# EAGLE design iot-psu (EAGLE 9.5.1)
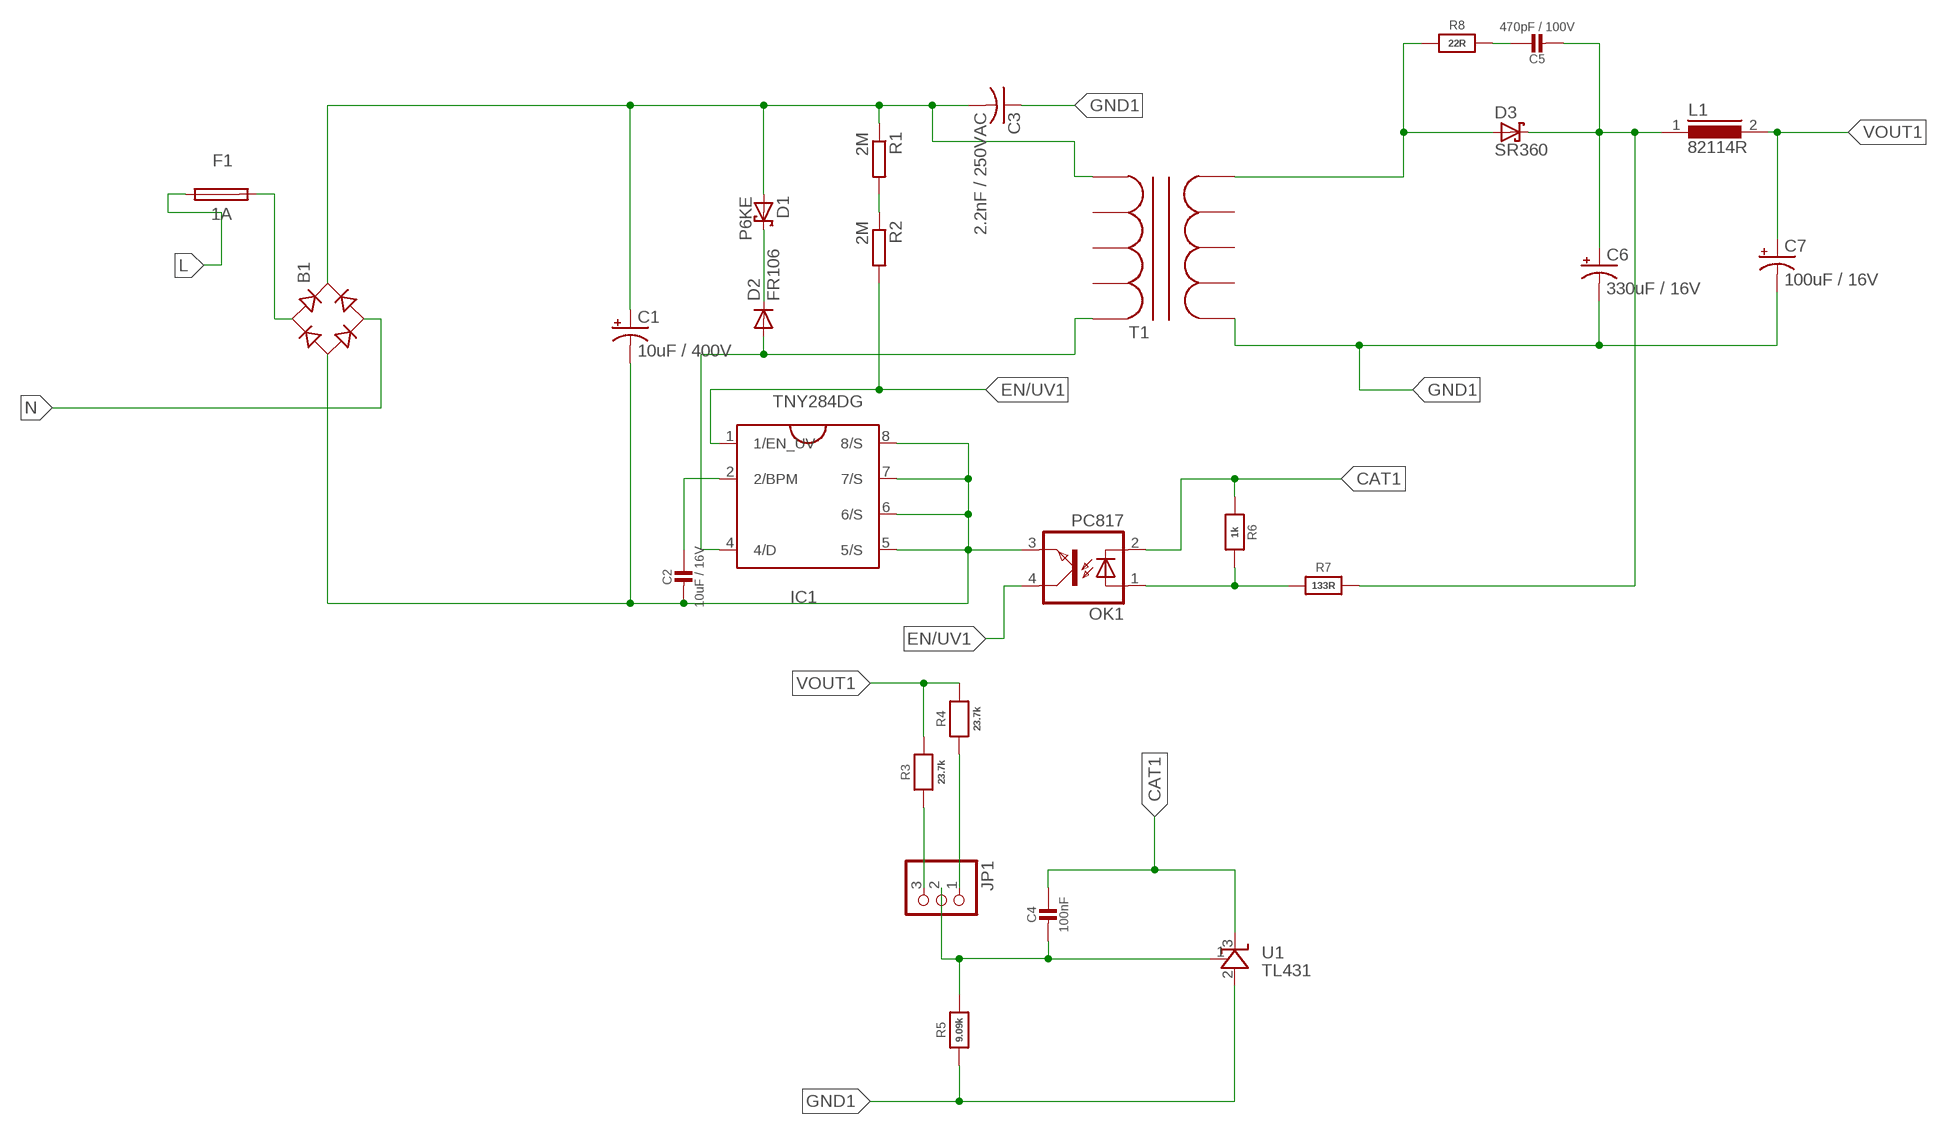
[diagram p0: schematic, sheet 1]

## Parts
B1  B-DIL  [B-DIL]
C1  10uF / 400V  CPOL-USE5-10.5  [E5-10,5]
C2  10uF / 16V  CAP_CERAMIC0805-NOOUTLINE  [0805-NO]
C3  2.2nF / 250VAC  C-US075-032X103  [C075-032X103]
C4  100nF  CAP_CERAMIC0805-NOOUTLINE  [0805-NO]
C5  470pF / 100V  CAP_CERAMIC0805-NOOUTLINE  [0805-NO]
C6  330uF / 16V  CPOL-USE3.5-8  [E3,5-8]
C7  100uF / 16V  CPOL-USE2.5-7  [E2,5-7]
D1  P6KE  P6KEXX  [CB417-15]
D2  FR106  1N4004  [DO41-10]
D3  SR360  SCHOTTKY-DIODEC4111-15  [C4111-15]
F1  1A  TR5  [TR5]
IC1  TNY284DG  TNY375-380SO8-C  [SO8-C(D_PACKAGE)]
JP1  PINHD-1X3  [1X03]
L1  82114R  [82114R]
OK1  PC817  [DIL04]
R1  2M  R-EU_M1206  [M1206]
R2  2M  R-EU_M1206  [M1206]
R3  23.7k  RESISTOR0805_NOOUTLINE  [0805-NO]
R4  23.7k  RESISTOR0805_NOOUTLINE  [0805-NO]
R5  9.09k  RESISTOR0805_NOOUTLINE  [0805-NO]
R6  1k  RESISTOR0805_NOOUTLINE  [0805-NO]
R7  133R  RESISTOR0805_NOOUTLINE  [0805-NO]
R8  22R  RESISTOR0805_NOOUTLINE  [0805-NO]
T1  TRANSFORMER_EE16  [EE16]
U1  TL431  [TO-92]

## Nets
AN1: C5.2 C6.+ D3.C L1.1 R7.2
BP/M: C2.1 IC1.2(2/BPM)
CAT1: C4.1 OK1.2(C) R6.1 U1.3(C)
DRAIN: D2.A IC1.4(4/D) T1.P$5
EN/UV1: IC1.1(1/EN_UV) OK1.4(COL) R2.2
GND1: C3.1 C6.- C7.- R5.1 T1.P$6 U1.2(A)
HV+: B1.+ C1.+ C3.2 D1.A R1.1 T1.P$1
L: F1.P$1
N: B1.AC2
N$1: JP1.1 R4.1
N$2: JP1.3 R3.1
N$5: OK1.1(A) R6.2 R7.1
N$6: D1.C D2.C
N$7: C5.1 R8.2
N$9: R1.2 R2.1
N$13: C4.2 JP1.2 R5.2 U1.1(REF)
N$50: B1.AC1 F1.P$2
SEC1: D3.A R8.1 T1.P$10
SOURCE: B1.- C1.- C2.2 IC1.5(5/S) IC1.6(6/S) IC1.7(7/S) IC1.8(8/S) OK1.3(EMIT)
VOUT1: C7.+ L1.2 R3.2 R4.2
Unconnected: T1.P$2 T1.P$3 T1.P$4 T1.P$7 T1.P$8 T1.P$9

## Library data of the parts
B1 = rectifier:B-DIL: RECTIFIER
C1 C6 C7 = resistor:CPOL-US: POLARIZED CAPACITOR, American symbol
C2 C4 C5 = microbuilder:CAP_CERAMIC: Ceramic Capacitors
C3 = resistor:C-US: CAPACITOR, American symbol
D1 = NRG Lib:P6KEXX: DIODE
D2 = NRG Lib:1N4004: DIODE
D3 = NRG Lib:SCHOTTKY-DIODE: Schottky Diode
F1 = nrg_single:TR5: FUSE
IC1 = power_integrations:TNY375-380: TinySwitch-PK incorporates a 700 V MOSFET, oscillator, highvoltage switched current source, current limit (user selectable), and thermal shutdown circuitry. A unique peak mode feature boosts current limit and frequency for peak load conditions. The boosted current limit provides the peak output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
JP1 = pinhead:PINHD-1X3: PIN HEADER
L1 = inductors:82114R: INDUCTOR
OK1 = NRG Lib:PC817: SHARP OPTO COUPLER; MPN: PC817X4J000F; OC_FARNELL: 9707727; OC_NEWARK: 97K7059
R1 R2 = resistor:R-EU_: RESISTOR, European symbol
R3-R8 = microbuilder:RESISTOR: Resistors
T1 = nrg_iso_rhythm:TRANSFORMER_EE16
U1 = NRG Lib:TL431

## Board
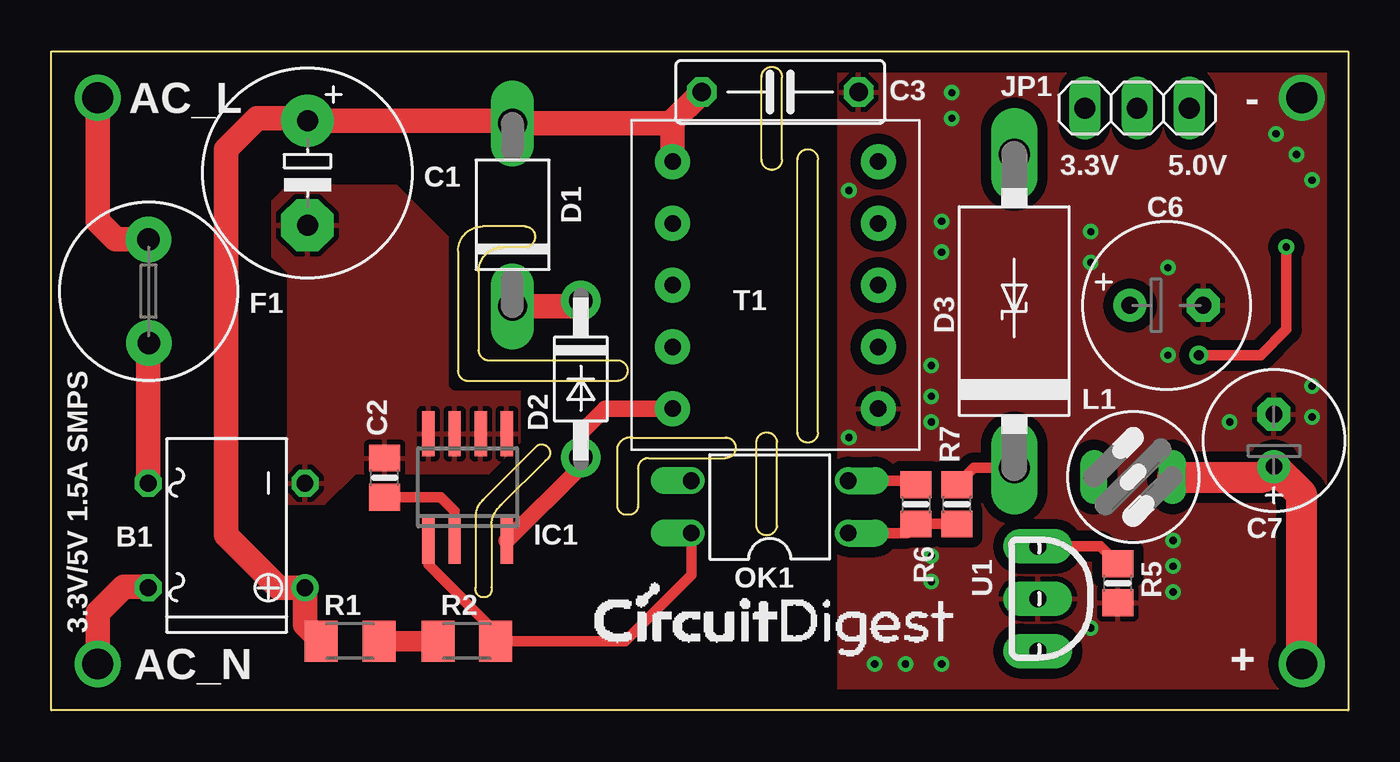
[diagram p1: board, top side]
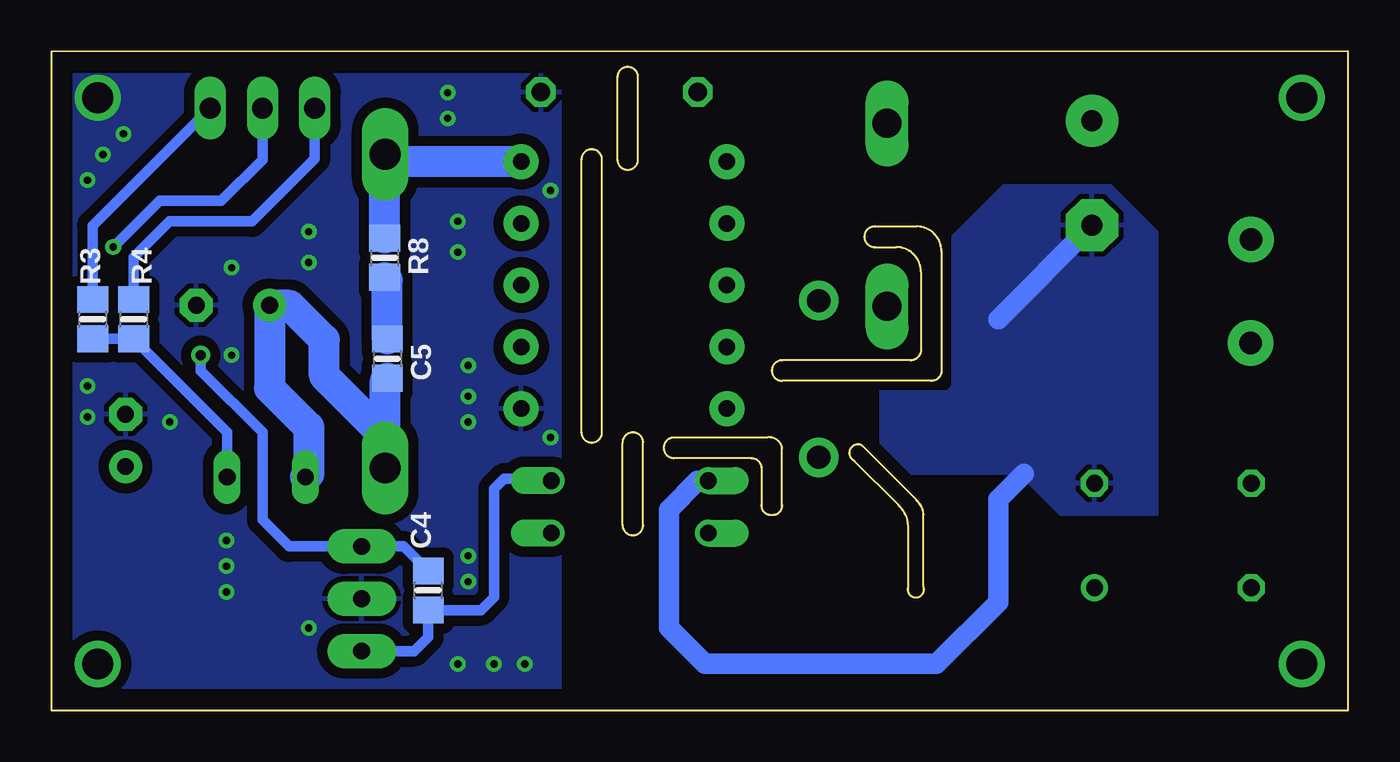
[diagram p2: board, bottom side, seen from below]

Size 63 x 32 mm. Coordinates in mm from the lower left corner, seen from the top.
Outline: 0,0 63,0 63,32 0,32 0,0
Copper layers (1*16): Top 0.035mm / dielectric 1.5mm / Bottom 0.035mm
Design rules "default *": minimum track width 6mil, minimum drill 0.35mm, track to track 0.35mm, track to pad 0.35mm, pad to pad 0.35mm, via to via 0.35mm, smd to smd 6mil, copper to edge 40mil, drill to drill 6mil, minimum pad ring 10mil, minimum via ring 8mil, stop-mask expansion 4mil, vias tented up to drill 0.5mm, thermal gap 10mil
Milling: 48 lines

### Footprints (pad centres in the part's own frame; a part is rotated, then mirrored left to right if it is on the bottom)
B-DIL = drill 0.813: + -2.54,-3.81 | drill 0.813 octagon: - 2.54,-3.81; AC1 2.54,3.81; AC2 -2.54,3.81
E5-10,5 = drill 1.016 pad 2.54: + -2.54,0 | drill 1.016 pad 2.54 octagon: - 2.54,0
0805-NO = smd 1.3 x 1.5: 1 -0.95,0; 2 0.95,0
C075-032X103 = drill 0.914 octagon: 1 -3.81,0; 2 3.81,0
E3,5-8 = drill 0.813 pad 1.6: + -1.778,0 | drill 0.813 pad 1.6 octagon: - 1.778,0
E2,5-7 = drill 0.813 pad 1.6: + -1.27,0 | drill 0.813 pad 1.6 octagon: - 1.27,0
CB417-15 = drill 1.397 long: A 2.54,0; C -6.35,0
DO41-10 = drill 1.118 pad 1.93: A 3.81,0; C -3.81,0
C4111-15 = drill 1.499 long: A 7.62,0; C -7.62,0
TR5 = drill 1.1 pad 2.2: P$1 -2.52,-0.01; P$2 2.51,0.02
SO8-C(D_PACKAGE) = smd 0.6 x 2.2: 1 -1.905,-2.6; 2 -0.635,-2.6; 4 1.905,-2.6; 5 1.905,2.6; 6 0.635,2.6; 7 -0.635,2.6; 8 -1.905,2.6
1X03 = drill 1.016 long: 1 -2.54,0; 2 0,0; 3 2.54,0
82114R = drill 0.813 long: 1 0,1.905; 2 0,-1.905
DIL04 = drill 0.813 offset: 1 -1.27,-3.81; 2 1.27,-3.81; 3 1.27,3.81; 4 -1.27,3.81
M1206 = smd 1.6 x 2: 1 -1.4,0; 2 1.4,0
EE16 = drill 0.8 pad 1.7: P$1 -6,-5; P$2 -3,-5; P$3 0,-5; P$4 3,-5; P$5 6,-5; P$6 6,5; P$7 3,5; P$8 0,5; P$9 -3,5; P$10 -6,5
TO-92 = drill 0.813 pad 1.676 long: 1 -2.54,0.318; 2 0,0.318; 3 2.54,0.318

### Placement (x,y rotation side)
B1  8.51,8.49 90 top
C1  12.44,26.1 270 top
C2  16.18,11.3 90 top
C3  35.41,30.03 180 top
C4  44.69,5.82 90 bottom
C5  46.68,17.08 270 bottom
C6  54.18,19.67 0 top
C7  59.4,13.11 90 top
D1  22.4,25.97 90 top
D2  25.72,16.09 270 top
D3  46.78,19.39 90 top
F1  4.72,20.35 270 top
IC1  20.22,10.83 0 top
JP1  52.75,29.25 0 top
L1  52.56,11.33 90 top
OK1  34.9,9.88 90 top
R1  14.51,3.36 0 top
R2  20.18,3.36 0 top
R3  61,19 270 bottom
R4  59,19 270 bottom
R5  51.81,6.17 90 top
R6  42,10 270 top
R7  44,10 90 top
R8  46.81,21.98 270 bottom
T1  35.18,20.65 270 top
U1  47.61,5.42 270 top

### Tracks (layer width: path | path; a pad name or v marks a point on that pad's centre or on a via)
AN1
  Top 0.5: R7.2 44.82,11.77 D3.C
  Bottom 1.5: L1.1 50.5,11.48 50.5,13.75 52.4,15.65 C6.+ 51.42,19.67 49.75,18 49.75,16.25 46.78,13.28 D3.C 46.78,16.03 C5.2
BP/M
  Top 0.5: IC1.2 19.59,9.66 18.9,10.35 C2.1
CAT1
  Top 0.5: OK1.2 41.8,11.15 R6.1
  Bottom 0.5: U1.3 45.37,2.88 44.69,3.56 C4.1 42.13,4.87 41.5,5.5 41.5,10.75 41,11.25 38.81,11.25 OK1.2
DRAIN
  Top 0.8: IC1.4 25.72,11.82 D2.A 25.72,13.47 26.9,14.65 T1.P$5
EN/UV1
  Top 0.5: IC1.1 18.32,7.07 21.58,3.8 R2.2 27.86,3.36 31.09,6.59 OK1.4
GND1  (via drill 0.35, 1.5)
  other vias: 60.75,29.75 42.75,16.75 42.75,15.25 42.75,14 50.5,4 43.25,2.25 41.5,2.25 40,2.25 38.75,13.25 42.75,6.25 42.75,7.5 54.5,8.25 54.5,7 54.5,5.75 61.25,14.25 61.25,15.75 57.25,14 54.25,17.25 54.25,21.5 50.5,23.25 50.5,21.75 43.25,23.75 43.25,22.25 59.5,28 60.5,27 61.25,25.75 43.75,30 43.75,28.75 38.75,25.25
  pour Bottom (isolate 0.5, rank 5): 38.25,31.5 62.5,31.5 62.5,0.5 38.25,0.5
  pour Top (isolate 0.5, rank 5): 38.25,31.5 62.5,31.5 62.5,1 38.25,1
HV+
  Top 1.2: R1.1 12.32,4.15 B1.+ 11.05,5.95 8.5,8.5 8.5,27.25 10,28.75 12.33,28.75 C1.+ 22.27,28.64 D1.A 30.08,28.51 | 30.08,28.51 C3.2 | T1.P$1 30.18,28.41 30.08,28.51
L  (via drill 1.5)
  Top 1.2: F1.P$1 3.13,22.87 2.25,23.75 v2.25,29.75
N  (via drill 1.5)
  Top 1.2: v2.25,2.25 2.25,4.75 3.5,6 4.65,6 B1.AC2
N$1
  Bottom 0.5: JP1.1 50.21,26.79 53.25,23.75 57.25,23.75 59,22 R4.1
N$2
  Bottom 0.5: JP1.3 61,23.54 R3.1
N$5
  Top 0.5: OK1.1 41.56,8.61 R6.2 R7.1
N$6
  Top 1.2: D1.C 25.44,19.62 D2.C
N$7
  Bottom 1.5: C5.1 46.68,20.9 R8.2
N$9
  Top 1: R1.2 R2.1
N$13  (via drill 0.35, 0.5)
  Top 0.5: R5.2 50.97,7.96 U1.1 | v55.75,17.25 58.75,17.25 60,18.5 v60,22.5
  Bottom 0.5: C4.2 45.88,7.96 U1.1 51.46,7.96 52.75,9.25 52.75,13.5 55.75,16.5 v55.75,17.25 | v60,22.5 57.75,24.75 54.75,24.75 52.75,26.75 JP1.2
N$50
  Top 1.2: B1.AC1 4.7,17.8 F1.P$2
SEC1
  Bottom 1.5: T1.P$10 46.42,26.65 | 46.42,26.65 D3.A | R8.1 46.81,26.26 46.42,26.65
SOURCE
  Bottom 1: OK1.3 31.6,11.15 33,9.75 33,4 31.25,2.25 20,2.25 17,5.25 17,10.25 15.75,11.5 | 17,19 C1.-
  pour Top: 10.75,22 10.75,24.75 11.5,25.5 16.75,25.5 19.25,23 19.25,15.75 19.5,15.5 22.75,15.5 22.75,13 21.25,11.5 14.75,11.5 13.25,10 11.5,10 11.5,21.25
  pour Bottom: 9.25,9.5 9.25,23.25 11.5,25.5 16.75,25.5 19.25,23 19.25,15.75 19.5,15.5 22.75,15.5 22.75,13 21.25,11.5 16,11.5 14,9.5
VOUT1  (via drill 1.5)
  Top 1.5: L1.2 58.89,11.33 C7.+ 60.75,10.49 v60.75,2.25
  Bottom 0.5: R3.2 R4.2 54.47,13.52 L1.2

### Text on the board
tNames: AC_L | - | 3.3V | 5.0V | 3.3V/5V 1.5A SMPS | AC_N | +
